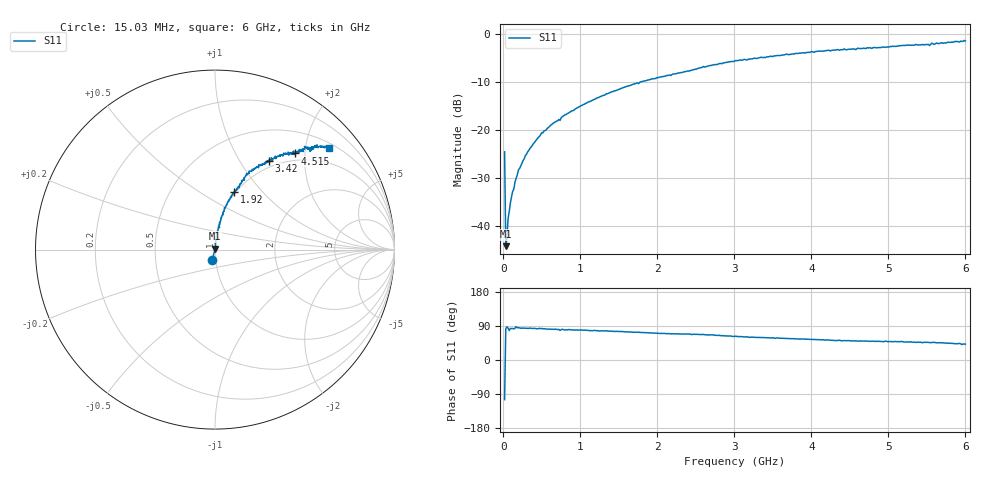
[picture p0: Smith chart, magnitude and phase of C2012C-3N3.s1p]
!	Network	Analyzer	HP8753E.07.74:	Oct	30	2002	Serial	No.	JP38451487
!	Hewlett-Packard
!	7	Sep	2009	10:38:55
!	Frequency	S11
#	HZ	S	RI	R	50
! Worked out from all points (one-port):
!   400 points, 15.03 MHz to 6 GHz, reference 50 ohm
!   lowest |S11| = -44.3 dB at 30.03 MHz (marker M1), VSWR 1.01, Z = 50.1 + j0.607 ohm
!   |S11| at or under -10 dB: start of sweep to 1.777 GHz
!   S11 on the Smith chart (normalised r, x): 15.03 MHz: 0.96, -0.11; 1.92 GHz: 0.98, +0.71; 3.42 GHz: 0.91, +1.35; 4.515 GHz: 0.86, +1.80; 6 GHz: 0.61, +2.49
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1.502992e7  -0.015 -0.0572
3.002985e7  0.000818 0.00606
4.502978e7  0.000304 0.00728
6.00297e7  0.00116 0.0118
9.002955e7  0.00207 0.0172
1.200294e8  0.00266 0.0227
1.95029e8  0.00303 0.0382
2.850286e8  0.00581 0.0539
4.950275e8  0.0106 0.0927
7.650262e8  0.0215 0.136
1.095025e9  0.0397 0.191
1.515022e9  0.0683 0.259
1.92002e9  0.107 0.321
2.265019e9  0.139 0.367
3.015015e9  0.243 0.472
3.420013e9  0.301 0.495
3.765011e9  0.345 0.517
4.515007e9  0.445 0.536
5.265004e9  0.52 0.566
5.535002e9  0.528 0.548
5.565002e9  0.56 0.58
5.595002e9  0.536 0.57
5.625002e9  0.57 0.575
5.715001e9  0.564 0.572
5.865001e9  0.617 0.573
5.925e9  0.595 0.575
5.955e9  0.639 0.549
6e9  0.633 0.566
